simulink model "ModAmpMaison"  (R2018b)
settings: Solver=ode45  StartTime=0.0  StopTime=10  RelTol=1e-3
libraries: simulink x1, dsparch4 x1, commrandsrc2 x1

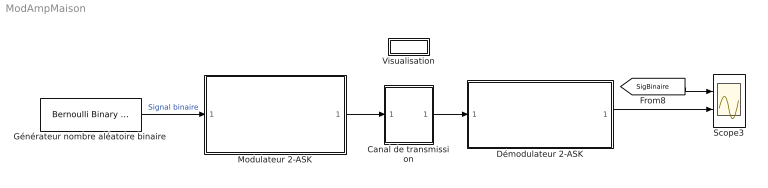
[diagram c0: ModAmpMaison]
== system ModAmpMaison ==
  Canal de transmission : Subsystem
  Démodulateur 2-ASK : Subsystem
  Générateur nombre aléatoire binaire : commrandsrc2/Bernoulli Binary Generator  P=0.4  seed=81  Ts=1  frameBased=off  sampPerFrame=1  orient=off  outDataType=double
  Modulateur 2-ASK : Subsystem
  Scope3 : Scope  NumInputPorts=2
  Visualisation : Subsystem
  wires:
  [SigBinaire] -> Scope3/1
  Générateur nombre aléatoire binaire/1 -> Modulateur 2-ASK/1(Signal binaire)  "Signal binaire"
  Modulateur 2-ASK/1(Signal Modulé ASK) -> Canal de transmission/1(In1)
  Démodulateur 2-ASK/1(Signal démodulé) -> Scope3/2
  Canal de transmission/1(Out1) -> Démodulateur 2-ASK/1(Signal modulé reçu)

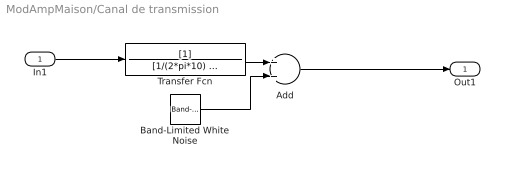
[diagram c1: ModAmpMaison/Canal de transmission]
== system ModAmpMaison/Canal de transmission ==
  In1 : Inport
  Add : Sum
  Band-Limited White Noise : simulink/Sources/Band-Limited White Noise  Cov=[0.002]  Ts=1  seed=[23341]
  Transfer Fcn : TransferFcn  Denominator=[1/(2*pi*10) 1]
  Out1 : Outport
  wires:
  Add/1 -> Out1/1
  Band-Limited White Noise/1 -> Add/2
  Transfer Fcn/1 -> Add/1
  In1/1 -> Transfer Fcn/1

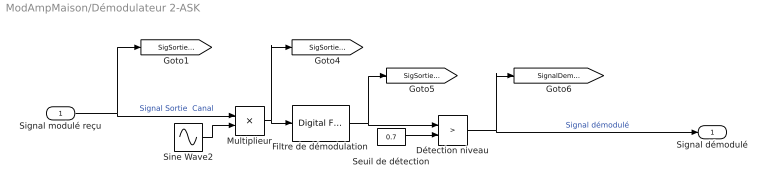
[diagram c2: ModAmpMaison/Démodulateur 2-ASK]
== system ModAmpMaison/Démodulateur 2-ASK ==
  Signal modulé reçu : Inport
  Détection niveau : RelationalOperator  Operator=>  OutDataTypeStr=boolean
  Filtre de démodulation : dsparch4/Digital Filter Design  mwdsp_browser_bugfix_var=off
  Multiplieur : Product
  Seuil de détection : Constant  Value=0.7
  Sine Wave2 : Sin  SineType=Sample based  Frequency=2*10*pi  Samples=50  SampleTime=1/200
  Signal démodulé : Outport
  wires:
  Filtre de démodulation/1 -> [SigSortieFiltre], Détection niveau/1
  Multiplieur/1 -> [SigSortieMult], Filtre de démodulation/1
  Seuil de détection/1 -> Détection niveau/2
  Sine Wave2/1 -> Multiplieur/2
  Détection niveau/1 -> Signal démodulé/1, [SignalDemodule]  "Signal démodulé"
  Signal modulé reçu/1 -> [SigSortieCanal], Multiplieur/1  "Signal Sortie  Canal"

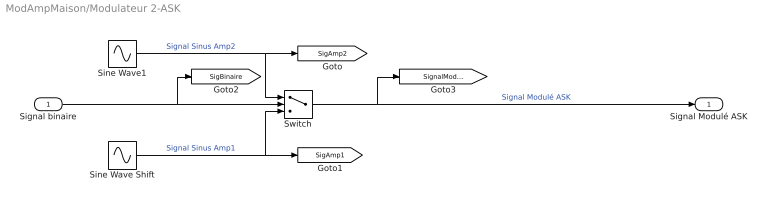
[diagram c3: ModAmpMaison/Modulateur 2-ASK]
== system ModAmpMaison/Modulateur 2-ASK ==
  Signal binaire : Inport
  Sine Wave Shift : Sin  SineType=Sample based  Frequency=2*10*pi  Phase=-pi  Samples=50  SampleTime=1/200
  Sine Wave1 : Sin  SineType=Sample based  Amplitude=2  Frequency=2*10*pi  Samples=50  SampleTime=1/200
  Switch : Switch  Threshold=0.5
  Signal Modulé ASK : Outport
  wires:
  Sine Wave1/1 -> [SigAmp2], Switch/1  "Signal Sinus Amp2"
  Switch/1 -> Signal Modulé ASK/1, [SignalModuleASK]  "Signal Modulé ASK"
  Sine Wave Shift/1 -> Switch/3, [SigAmp1]  "Signal Sinus Amp1"
  Signal binaire/1 -> [SigBinaire], Switch/2

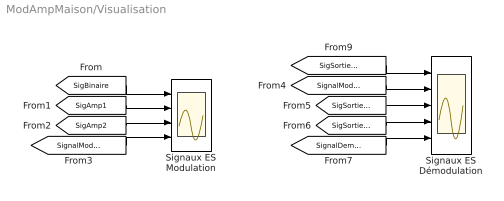
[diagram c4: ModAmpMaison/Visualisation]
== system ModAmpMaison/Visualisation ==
  Signaux ES Démodulation : Scope  NumInputPorts=5
  Signaux ES Modulation : Scope  NumInputPorts=4
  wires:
  [SignalModuleASK] -> Signaux ES Démodulation/2
  [SigSortieFiltre] -> Signaux ES Démodulation/4
  [SigBinaire] -> Signaux ES Modulation/1
  [SigAmp1] -> Signaux ES Modulation/2
  [SignalModuleASK] -> Signaux ES Modulation/4
  [SigSortieCanal] -> Signaux ES Démodulation/1
  [SignalDemodule] -> Signaux ES Démodulation/5
  [SigSortieMult] -> Signaux ES Démodulation/3
  [SigAmp2] -> Signaux ES Modulation/3
